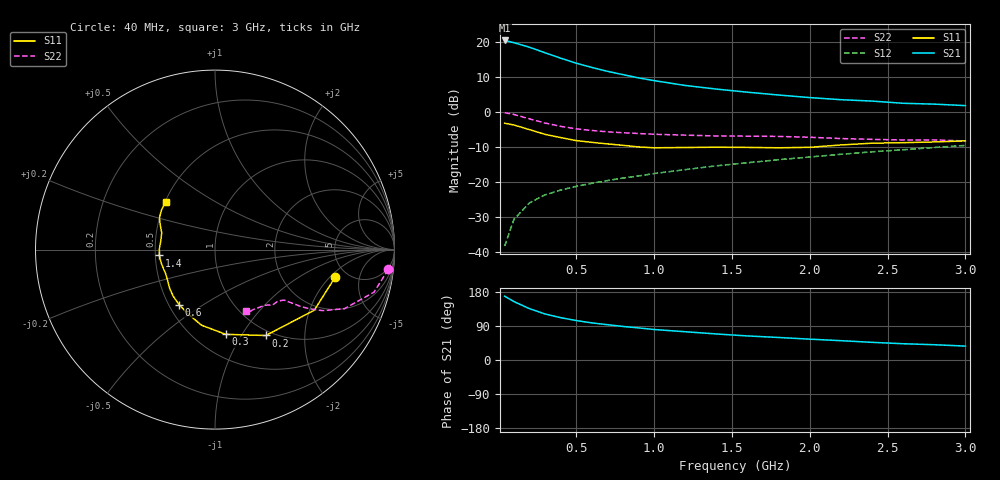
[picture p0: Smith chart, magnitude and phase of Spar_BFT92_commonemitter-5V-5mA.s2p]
! Filename:  BFT92B.S2P  Version:  2.0
! NXP part #: BFT92  Date: May 1990
! Bias condition: Vce=-5V, Ic=-5mA
#  MHz  S  MA  R  50
! Freq  S11  S21  S12  S22  !GUM [dB]
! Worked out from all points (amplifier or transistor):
!   21 points, 40 MHz to 3 GHz, reference 50 ohm
!   highest |S21| = 20.4 dB at 40 MHz (marker M1)
!   |S21| within 3 dB of that: start of sweep to 266.8 MHz
!   unconditionally stable (mu >= 1): 971 MHz to 2.674 GHz
!   at 300 MHz: K = 0.54, MSG = 20.3 dB, |S12| = -23.7 dB
!   at 1 GHz: K = 1.01, MAG = 12.7 dB, |S12| = -17.7 dB
!   at 3 GHz: K = 0.97, MSG = 5.7 dB, |S12| = -9.6 dB
!   S11 on the Smith chart (normalised r, x): 40 MHz: 3.98, -2.31; 200 MHz: 0.93, -1.29; 300 MHz: 0.70, -0.85; 600 MHz: 0.56, -0.40; 1.4 GHz: 0.53, -0.04; 3 GHz: 0.50, +0.32
40  0.687 -12.9  10.48 168.4  0.012 83.2  0.972 -6.5
100  0.648 -31.4  9.739 154.2  0.029 73.9  0.917 -15.0
200  0.556 -59.4  8.379 135.4  0.05 65.0  0.793 -24.5
300  0.476 -82.7  6.984 121.4  0.065 60.6  0.691 -29.5
400  0.428 -100.1  5.849 111.7  0.076 58.8  0.62 -32.1
500  0.388 -112.9  4.956 104.1  0.086 58.4  0.571 -33.6
600  0.366 -123.3  4.314 97.9  0.095 58.9  0.541 -34.3
700  0.348 -132.2  3.795 93.2  0.104 59.7  0.518 -34.9
800  0.332 -139.6  3.403 88.6  0.113 60.6  0.502 -35.4
900  0.315 -147.0  3.056 84.6  0.121 61.3  0.49 -35.7
1000  0.306 -153.6  2.795 80.5  0.131 62.0  0.478 -36.1
1200  0.309 -166.0  2.381 74.6  0.149 63.0  0.464 -37.7
1400  0.312 -174.0  2.115 68.7  0.169 63.7  0.452 -39.9
1600  0.31 179.1  1.909 63.5  0.187 64.1  0.449 -41.7
1800  0.306 171.5  1.738 59.4  0.207 64.6  0.445 -43.8
2000  0.311 162.7  1.598 55.0  0.226 64.6  0.433 -45.5
2200  0.336 155.3  1.491 51.0  0.247 64.6  0.415 -48.3
2400  0.356 150.4  1.424 46.6  0.268 63.8  0.404 -53.2
2600  0.362 147.6  1.325 42.9  0.287 63.4  0.396 -57.5
2800  0.371 143.5  1.288 40.3  0.309 63.2  0.397 -60.5
3000  0.384 135.8  1.227 36.7  0.331 62.5  0.383 -63.2
